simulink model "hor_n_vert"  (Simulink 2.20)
settings: Solver=ode1  StartTime=0.0  StopTime=1  FixedStep=0.001  MaxStep=0.001  RelTol=1e-5  AbsTol=1e-5
undefined symbols (not defined in the file or in its folder): sfuny
libraries: simulink x1

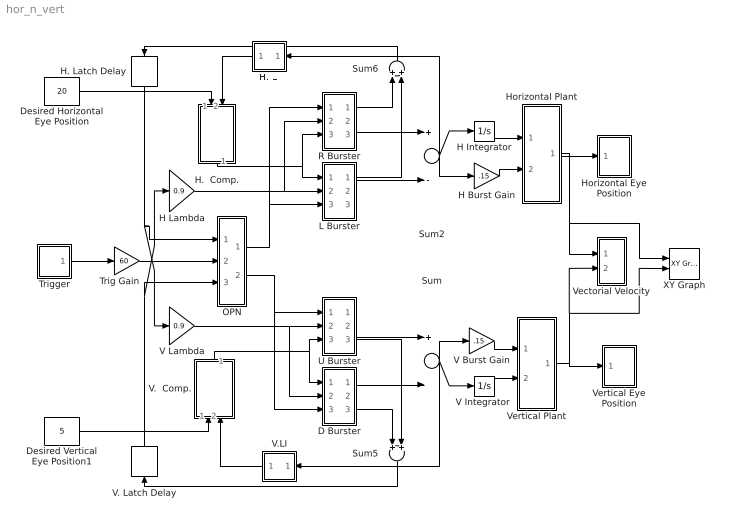
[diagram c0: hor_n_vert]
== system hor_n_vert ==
  D Burster : Subsystem
  Desired Horizontal Eye Position : Constant  Value=20
  Desired Vertical Eye Position1 : Constant  Value=5
  H Burst Gain : Gain  Gain=.15
  H Integrator : Integrator  ExternalReset=none  InitialConditionSource=internal  InitialCondition=0  LimitOutput=off  UpperSaturationLimit=inf  LowerSaturationLimit=-inf  ShowSaturationPort=off  ShowStatePort=off  AbsoluteTolerance=auto
  H Lambda : Gain  Gain=0.9
  H.  Comp. : Subsystem  Orientation=down
  H. LI : Subsystem  Orientation=left
  H. Latch Delay : TransportDelay  Orientation=down  DelayTime=.001  InitialInput=00  BufferSize=1024
  Horizontal Plant : Subsystem
  Horizontal Eye Position : Subsystem  LoadFcn=sfuny([],[],[],'LoadBlock')  StartFcn=sfuny([],[],[],'Start')  StopFcn=sfuny([],[],[],'Stop')  mask(Graph scope.){}
      mask help: Graph scope using MATLAB graph window. Enter plotting ranges and line type.
      mask init:
      | color = @4; ax = [0, @1, @2, @3]; dt = -1;
  L Burster : Subsystem
  OPN : Subsystem
  R Burster : Subsystem
  Sum : Sum  Inputs=+-
  Sum2 : Sum  Inputs=+-
  Sum5 : Sum  Orientation=down  Inputs=++
  Sum6 : Sum  Orientation=up  Inputs=++
  Trig Gain : Gain  Gain=60
  Trigger : Subsystem  mask(Pulse Generator){period=1, duty=3, amplitude=1, start=.1}
      mask prompts: period "Period (secs):"; duty "Duty cycle (% of period):"; start "Start time:"
      mask help: Pulse Generator
  U Burster : Subsystem
  V Burst Gain : Gain  Gain=.15
  "V Integrator " : Integrator  ExternalReset=none  InitialConditionSource=internal  InitialCondition=0  LimitOutput=off  UpperSaturationLimit=inf  LowerSaturationLimit=-inf  ShowSaturationPort=off  ShowStatePort=off  AbsoluteTolerance=auto
  V Lambda : Gain  Gain=0.9
  V.  Comp. : Subsystem  Orientation=up
  V. Latch Delay : TransportDelay  Orientation=up  DelayTime=.001  InitialInput=00  BufferSize=1024
  V.LI : Subsystem  Orientation=left
  Vectorial Velocity : Subsystem
  Vertical Plant : Subsystem
  Vertical Eye Position : Subsystem  LoadFcn=sfuny([],[],[],'LoadBlock')  StartFcn=sfuny([],[],[],'Start')  StopFcn=sfuny([],[],[],'Stop')  mask(Graph scope.){}
      mask help: Graph scope using MATLAB graph window. Enter plotting ranges and line type.
      mask init:
      | color = @4; ax = [0, @1, @2, @3]; dt = -1;
  XY Graph : simulink/Sinks/XY Graph  xmin=-25  xmax=25  ymin=-25  ymax=25  st=-1
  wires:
  Horizontal Plant/1(out_1) -> Horizontal Eye Position/1(x), Vectorial Velocity/1(Horizontal Position), XY Graph/1
  H Integrator/1 -> Horizontal Plant/1(in_1)
  OPN/2(out_4) -> D Burster/3(in_3), U Burster/1(in_3)
  OPN/1(out_1) -> R Burster/1(in_3), L Burster/3(in_3)
  H. Latch Delay/1 -> V Lambda/1, OPN/1(in_1)
  V. Latch Delay/1 -> H Lambda/1, OPN/3(in_3)
  Trig Gain/1 -> OPN/2(in_2)
  R Burster/1(out_2) -> Sum6/1
  V.LI/1(out_1) -> V.  Comp./2(in_5)
  H. LI/1(out_1) -> H.  Comp./2(in_2)
  Sum5/1 -> V. Latch Delay/1
  Sum6/1 -> H. Latch Delay/1
  L Burster/1(out_1) -> Sum6/2
  V.  Comp./1(out_1) -> D Burster/1(in_1), U Burster/3(in_1)
  V Lambda/1 -> D Burster/2(in_2), U Burster/2(in_2)
  D Burster/2(out_2) -> Sum/2
  D Burster/3(out_3) -> Sum5/1
  U Burster/2(out_3) -> Sum/1
  U Burster/3(out_4) -> Sum5/2
  H Lambda/1 -> R Burster/2(in_2), L Burster/2(in_2)
  R Burster/2(out_3) -> Sum2/1
  L Burster/2(out_2) -> Sum2/2
  H.  Comp./1(out_1) -> R Burster/3(in_1), L Burster/1(in_1)
  Sum/1 -> V.LI/1(in_1), "V Integrator "/1, V Burst Gain/1
  "V Integrator "/1 -> Vertical Plant/2(in_2)
  V Burst Gain/1 -> Vertical Plant/1(in_1)
  Sum2/1 -> H. LI/1(in_1), H Burst Gain/1, H Integrator/1
  H Burst Gain/1 -> Horizontal Plant/2(in_2)
  Vertical Plant/1(out_1) -> Vertical Eye Position/1(x), Vectorial Velocity/2(Veritcal Position), XY Graph/2
  Trigger/1(out1) -> Trig Gain/1
  Desired Horizontal Eye Position/1 -> H.  Comp./1(in_1)
  Desired Vertical Eye Position1/1 -> V.  Comp./1(in_4)

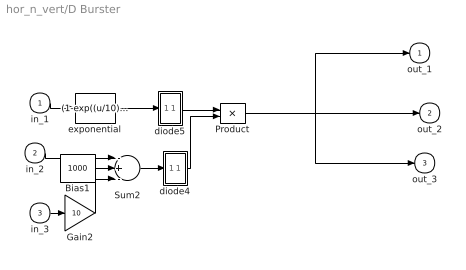
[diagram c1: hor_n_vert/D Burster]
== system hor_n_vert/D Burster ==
  in_1 : Inport  Port=1  PortWidth=-1  SampleTime=-1
  in_2 : Inport  Port=2  PortWidth=-1  SampleTime=-1
  in_3 : Inport  Port=3  PortWidth=-1  SampleTime=-1
  Bias1 : Constant  Value=1000
  Gain2 : Gain  Gain=10
  Product : Product  Inputs=2
  Sum2 : Sum  Inputs=-+-
  diode4 : Subsystem
  diode5 : Subsystem
  exponential : Fcn  Expr=(1-exp((u/10)))
  out_1 : Outport  Port=1  InitialOutput=0
  out_2 : Outport  Port=2  InitialOutput=0
  out_3 : Outport  Port=3  InitialOutput=0
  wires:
  in_1/1 -> exponential/1
  Bias1/1 -> Sum2/2
  in_2/1 -> Sum2/1
  in_3/1 -> Gain2/1
  Gain2/1 -> Sum2/3
  Sum2/1 -> diode4/1(in_1)
  diode4/1(out_1) -> Product/2
  exponential/1 -> diode5/1(in_1)
  diode5/1(out_1) -> Product/1
  Product/1 -> out_1/1, out_2/1, out_3/1

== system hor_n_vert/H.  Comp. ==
  in_1 : Inport  Port=1  PortWidth=-1  SampleTime=-1
  in_2 : Inport  Port=2  PortWidth=-1  SampleTime=-1
  Sum : Sum  Inputs=+-
  out_1 : Outport  Port=1  InitialOutput=0
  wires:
  in_2/1 -> Sum/2
  in_1/1 -> Sum/1
  Sum/1 -> out_1/1

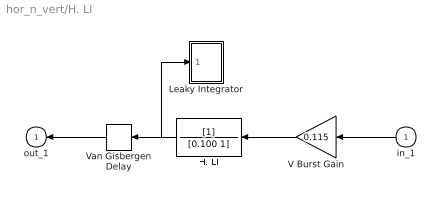
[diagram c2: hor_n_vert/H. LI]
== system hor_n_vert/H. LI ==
  in_1 : Inport  Orientation=left  Port=1  PortWidth=-1  SampleTime=-1
  H. LI : TransferFcn  Orientation=left  Numerator=[1]  Denominator=[0.100 1]
  Leaky Integrator : Subsystem  LoadFcn=sfuny([],[],[],'LoadBlock')  StartFcn=sfuny([],[],[],'Start')  StopFcn=sfuny([],[],[],'Stop')  mask(Graph scope.){}
      mask help: Graph scope using MATLAB graph window. Enter plotting ranges and line type.
      mask init:
      | color = @4; ax = [0, @1, @2, @3]; dt = -1;
  V Burst Gain : Gain  Orientation=left  Gain=0.115
  Van Gisbergen Delay : TransportDelay  Orientation=left  DelayTime=.002  InitialInput=00  BufferSize=1024
  out_1 : Outport  Orientation=left  Port=1  InitialOutput=0
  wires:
  Van Gisbergen Delay/1 -> out_1/1
  in_1/1 -> V Burst Gain/1
  V Burst Gain/1 -> H. LI/1
  H. LI/1 -> Van Gisbergen Delay/1, Leaky Integrator/1(x)

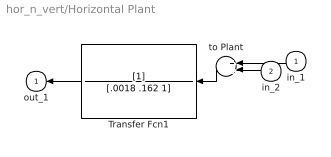
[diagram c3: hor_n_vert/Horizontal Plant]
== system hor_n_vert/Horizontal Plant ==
  in_1 : Inport  Orientation=left  Port=1  PortWidth=-1  SampleTime=-1
  in_2 : Inport  Orientation=left  Port=2  PortWidth=-1  SampleTime=-1
  Transfer Fcn1 : TransferFcn  Orientation=left  Numerator=[1]  Denominator=[.0018 .162 1]
  to Plant : Sum  Orientation=left  Inputs=++
  out_1 : Outport  Orientation=left  Port=1  InitialOutput=0
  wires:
  Transfer Fcn1/1 -> out_1/1
  in_2/1 -> to Plant/2
  in_1/1 -> to Plant/1
  to Plant/1 -> Transfer Fcn1/1

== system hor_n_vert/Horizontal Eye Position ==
  x : Inport  Port=1  PortWidth=-1  SampleTime=-1
  "S-function M-file which plots lines " : S-Function  FunctionName=sfuny  Parameters=ax, color,dt  PortCounts=[]  SFunctionModules=''
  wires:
  x/1 -> "S-function M-file which plots lines "/1

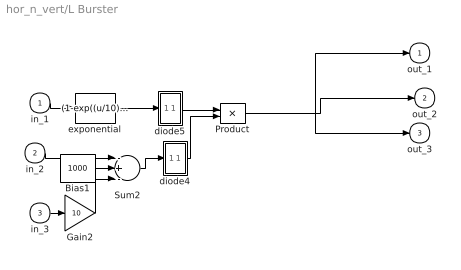
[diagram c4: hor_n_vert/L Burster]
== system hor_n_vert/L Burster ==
  in_1 : Inport  Port=1  PortWidth=-1  SampleTime=-1
  in_2 : Inport  Port=2  PortWidth=-1  SampleTime=-1
  in_3 : Inport  Port=3  PortWidth=-1  SampleTime=-1
  Bias1 : Constant  Value=1000
  Gain2 : Gain  Gain=10
  Product : Product  Inputs=2
  Sum2 : Sum  Inputs=-+-
  diode4 : Subsystem
  diode5 : Subsystem
  exponential : Fcn  Expr=(1-exp((u/10)))
  out_1 : Outport  Port=1  InitialOutput=0
  out_2 : Outport  Port=2  InitialOutput=0
  out_3 : Outport  Port=3  InitialOutput=0
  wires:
  Product/1 -> out_3/1, out_2/1, out_1/1
  diode5/1(out_1) -> Product/1
  exponential/1 -> diode5/1(in_1)
  diode4/1(out_1) -> Product/2
  Sum2/1 -> diode4/1(in_1)
  Gain2/1 -> Sum2/3
  in_3/1 -> Gain2/1
  in_2/1 -> Sum2/1
  Bias1/1 -> Sum2/2
  in_1/1 -> exponential/1

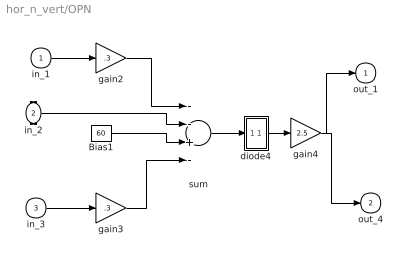
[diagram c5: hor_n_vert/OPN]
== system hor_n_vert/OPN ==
  in_1 : Inport  Port=1  PortWidth=-1  SampleTime=-1
  in_2 : Inport  Port=2  PortWidth=-1  SampleTime=-1
  in_3 : Inport  Port=3  PortWidth=-1  SampleTime=-1
  Bias1 : Constant  Value=60
  diode4 : Subsystem
  gain2 : Gain  Gain=.3
  gain3 : Gain  Gain=.3
  gain4 : Gain  Gain=2.5
  sum : Sum  Inputs=--+-
  out_1 : Outport  Port=1  InitialOutput=0
  out_4 : Outport  Port=2  InitialOutput=0
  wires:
  gain4/1 -> out_4/1, out_1/1
  diode4/1(out_1) -> gain4/1
  gain3/1 -> sum/4
  in_3/1 -> gain3/1
  gain2/1 -> sum/1
  in_1/1 -> gain2/1
  Bias1/1 -> sum/3
  in_2/1 -> sum/2
  sum/1 -> diode4/1(in_1)

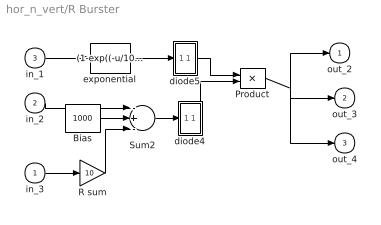
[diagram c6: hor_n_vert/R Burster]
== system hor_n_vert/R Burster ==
  in_3 : Inport  Port=1  PortWidth=-1  SampleTime=-1
  in_2 : Inport  Port=2  PortWidth=-1  SampleTime=-1
  in_1 : Inport  Port=3  PortWidth=-1  SampleTime=-1
  Bias : Constant  Value=1000
  Product : Product  Inputs=2
  R sum : Gain  Gain=10
  Sum2 : Sum  Inputs=-+-
  diode4 : Subsystem
  diode5 : Subsystem
  exponential : Fcn  Expr=(1-exp((-u/10)))
  out_2 : Outport  Port=1  InitialOutput=0
  out_3 : Outport  Port=2  InitialOutput=0
  out_4 : Outport  Port=3  InitialOutput=0
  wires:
  diode5/1(out_1) -> Product/1
  exponential/1 -> diode5/1(in_1)
  diode4/1(out_1) -> Product/2
  Sum2/1 -> diode4/1(in_1)
  in_1/1 -> exponential/1
  in_2/1 -> Sum2/1
  Bias/1 -> Sum2/2
  Product/1 -> out_2/1, out_4/1, out_3/1
  in_3/1 -> R sum/1
  R sum/1 -> Sum2/3

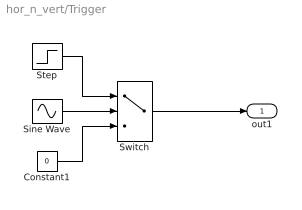
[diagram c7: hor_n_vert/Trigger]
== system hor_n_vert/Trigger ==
  Constant1 : Constant  Value=0
  Sine Wave : Sin  Amplitude=1  Frequency=2*pi./period  Phase=-2*pi*(start./period + duty/200 - 1/4)  SampleTime=-1
  Step : Step  Time=start  Before=0  After=amplitude
  Switch : Switch  Threshold=sin(pi*(0.5 - duty/100))
  out1 : Outport  Port=1  InitialOutput=0
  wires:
  Sine Wave/1 -> Switch/2
  Switch/1 -> out1/1
  Constant1/1 -> Switch/3
  Step/1 -> Switch/1

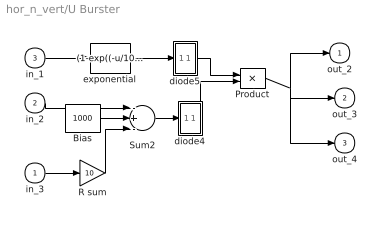
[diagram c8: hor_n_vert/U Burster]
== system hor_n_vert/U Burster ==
  in_3 : Inport  Port=1  PortWidth=-1  SampleTime=-1
  in_2 : Inport  Port=2  PortWidth=-1  SampleTime=-1
  in_1 : Inport  Port=3  PortWidth=-1  SampleTime=-1
  Bias : Constant  Value=1000
  Product : Product  Inputs=2
  R sum : Gain  Gain=10
  Sum2 : Sum  Inputs=-+-
  diode4 : Subsystem
  diode5 : Subsystem
  exponential : Fcn  Expr=(1-exp((-u/10)))
  out_2 : Outport  Port=1  InitialOutput=0
  out_3 : Outport  Port=2  InitialOutput=0
  out_4 : Outport  Port=3  InitialOutput=0
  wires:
  diode5/1(out_1) -> Product/1
  exponential/1 -> diode5/1(in_1)
  diode4/1(out_1) -> Product/2
  Sum2/1 -> diode4/1(in_1)
  in_1/1 -> exponential/1
  in_2/1 -> Sum2/1
  Bias/1 -> Sum2/2
  Product/1 -> out_2/1, out_4/1, out_3/1
  in_3/1 -> R sum/1
  R sum/1 -> Sum2/3

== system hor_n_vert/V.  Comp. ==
  in_4 : Inport  Port=1  PortWidth=-1  SampleTime=-1
  in_5 : Inport  Port=2  PortWidth=-1  SampleTime=-1
  Sum : Sum  Inputs=-+
  out_1 : Outport  Port=1  InitialOutput=0
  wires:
  in_4/1 -> Sum/2
  in_5/1 -> Sum/1
  Sum/1 -> out_1/1

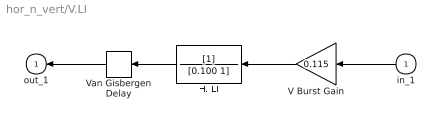
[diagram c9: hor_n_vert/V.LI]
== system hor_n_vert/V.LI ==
  in_1 : Inport  Orientation=left  Port=1  PortWidth=-1  SampleTime=-1
  H. LI : TransferFcn  Orientation=left  Numerator=[1]  Denominator=[0.100 1]
  V Burst Gain : Gain  Orientation=left  Gain=0.115
  Van Gisbergen Delay : TransportDelay  Orientation=left  DelayTime=.002  InitialInput=00  BufferSize=1024
  out_1 : Outport  Orientation=left  Port=1  InitialOutput=0
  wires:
  H. LI/1 -> Van Gisbergen Delay/1
  V Burst Gain/1 -> H. LI/1
  in_1/1 -> V Burst Gain/1
  Van Gisbergen Delay/1 -> out_1/1

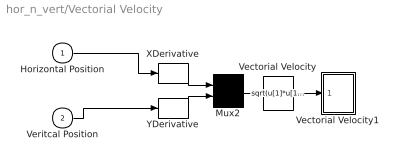
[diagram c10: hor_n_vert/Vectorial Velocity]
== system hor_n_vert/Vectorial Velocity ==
  Horizontal Position : Inport  Port=1  PortWidth=-1  SampleTime=-1
  Veritcal Position : Inport  Port=2  PortWidth=-1  SampleTime=-1
  Mux2 : Mux  Inputs=2
  Vectorial Velocity : Fcn  Expr=sqrt(u[1]*u[1]+u[2]*u[2])
  Vectorial Velocity1 : Subsystem  LoadFcn=sfuny([],[],[],'LoadBlock')  StartFcn=sfuny([],[],[],'Start')  StopFcn=sfuny([],[],[],'Stop')  mask(Graph scope.){}
      mask help: Graph scope using MATLAB graph window. Enter plotting ranges and line type.
      mask init:
      | color = @4; ax = [0, @1, @2, @3]; dt = -1;
  XDerivative : Derivative
  YDerivative : Derivative
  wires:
  Veritcal Position/1 -> YDerivative/1
  Horizontal Position/1 -> XDerivative/1
  Mux2/1 -> Vectorial Velocity/1
  XDerivative/1 -> Mux2/1
  YDerivative/1 -> Mux2/2
  Vectorial Velocity/1 -> Vectorial Velocity1/1(x)

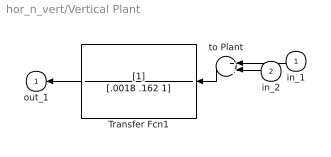
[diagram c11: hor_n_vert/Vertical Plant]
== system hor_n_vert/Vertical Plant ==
  in_1 : Inport  Orientation=left  Port=1  PortWidth=-1  SampleTime=-1
  in_2 : Inport  Orientation=left  Port=2  PortWidth=-1  SampleTime=-1
  Transfer Fcn1 : TransferFcn  Orientation=left  Numerator=[1]  Denominator=[.0018 .162 1]
  to Plant : Sum  Orientation=left  Inputs=++
  out_1 : Outport  Orientation=left  Port=1  InitialOutput=0
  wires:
  Transfer Fcn1/1 -> out_1/1
  in_2/1 -> to Plant/2
  in_1/1 -> to Plant/1
  to Plant/1 -> Transfer Fcn1/1

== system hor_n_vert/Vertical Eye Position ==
  x : Inport  Port=1  PortWidth=-1  SampleTime=-1
  "S-function M-file which plots lines " : S-Function  FunctionName=sfuny  Parameters=ax, color,dt  PortCounts=[]  SFunctionModules=''
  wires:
  x/1 -> "S-function M-file which plots lines "/1

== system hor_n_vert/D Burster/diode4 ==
  in_1 : Inport  Port=1  PortWidth=-1  SampleTime=-1
  Switch : Switch  Threshold=0
  diode1 : Constant  Value=0
  out_1 : Outport  Port=1  InitialOutput=0
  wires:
  in_1/1 -> Switch/2, Switch/1
  Switch/1 -> out_1/1
  diode1/1 -> Switch/3

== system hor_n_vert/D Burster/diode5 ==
  in_1 : Inport  Port=1  PortWidth=-1  SampleTime=-1
  Switch : Switch  Threshold=0
  diode1 : Constant  Value=0
  out_1 : Outport  Port=1  InitialOutput=0
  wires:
  in_1/1 -> Switch/2, Switch/1
  Switch/1 -> out_1/1
  diode1/1 -> Switch/3

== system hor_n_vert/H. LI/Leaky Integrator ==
  x : Inport  Port=1  PortWidth=-1  SampleTime=-1
  "S-function M-file which plots lines " : S-Function  FunctionName=sfuny  Parameters=ax, color,dt  PortCounts=[]  SFunctionModules=''
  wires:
  x/1 -> "S-function M-file which plots lines "/1

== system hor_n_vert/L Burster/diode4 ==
  in_1 : Inport  Port=1  PortWidth=-1  SampleTime=-1
  Switch : Switch  Threshold=0
  diode1 : Constant  Value=0
  out_1 : Outport  Port=1  InitialOutput=0
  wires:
  diode1/1 -> Switch/3
  Switch/1 -> out_1/1
  in_1/1 -> Switch/2, Switch/1

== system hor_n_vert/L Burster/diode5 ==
  in_1 : Inport  Port=1  PortWidth=-1  SampleTime=-1
  Switch : Switch  Threshold=0
  diode1 : Constant  Value=0
  out_1 : Outport  Port=1  InitialOutput=0
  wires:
  diode1/1 -> Switch/3
  Switch/1 -> out_1/1
  in_1/1 -> Switch/2, Switch/1

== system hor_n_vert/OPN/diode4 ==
  in_1 : Inport  Port=1  PortWidth=-1  SampleTime=-1
  Switch : Switch  Threshold=0
  diode1 : Constant  Value=0
  out_1 : Outport  Port=1  InitialOutput=0
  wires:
  in_1/1 -> Switch/2, Switch/1
  Switch/1 -> out_1/1
  diode1/1 -> Switch/3

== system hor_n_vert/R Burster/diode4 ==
  in_1 : Inport  Port=1  PortWidth=-1  SampleTime=-1
  Switch : Switch  Threshold=0
  diode1 : Constant  Value=0
  out_1 : Outport  Port=1  InitialOutput=0
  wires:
  in_1/1 -> Switch/2, Switch/1
  Switch/1 -> out_1/1
  diode1/1 -> Switch/3

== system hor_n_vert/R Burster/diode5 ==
  in_1 : Inport  Port=1  PortWidth=-1  SampleTime=-1
  Switch : Switch  Threshold=0
  diode1 : Constant  Value=0
  out_1 : Outport  Port=1  InitialOutput=0
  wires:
  diode1/1 -> Switch/3
  Switch/1 -> out_1/1
  in_1/1 -> Switch/2, Switch/1

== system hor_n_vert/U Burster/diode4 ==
  in_1 : Inport  Port=1  PortWidth=-1  SampleTime=-1
  Switch : Switch  Threshold=0
  diode1 : Constant  Value=0
  out_1 : Outport  Port=1  InitialOutput=0
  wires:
  in_1/1 -> Switch/2, Switch/1
  Switch/1 -> out_1/1
  diode1/1 -> Switch/3

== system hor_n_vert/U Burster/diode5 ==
  in_1 : Inport  Port=1  PortWidth=-1  SampleTime=-1
  Switch : Switch  Threshold=0
  diode1 : Constant  Value=0
  out_1 : Outport  Port=1  InitialOutput=0
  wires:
  diode1/1 -> Switch/3
  Switch/1 -> out_1/1
  in_1/1 -> Switch/2, Switch/1

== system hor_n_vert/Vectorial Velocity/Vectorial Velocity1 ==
  x : Inport  Port=1  PortWidth=-1  SampleTime=-1
  "S-function M-file which plots lines " : S-Function  FunctionName=sfuny  Parameters=ax, color,dt  PortCounts=[]  SFunctionModules=''
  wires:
  x/1 -> "S-function M-file which plots lines "/1
